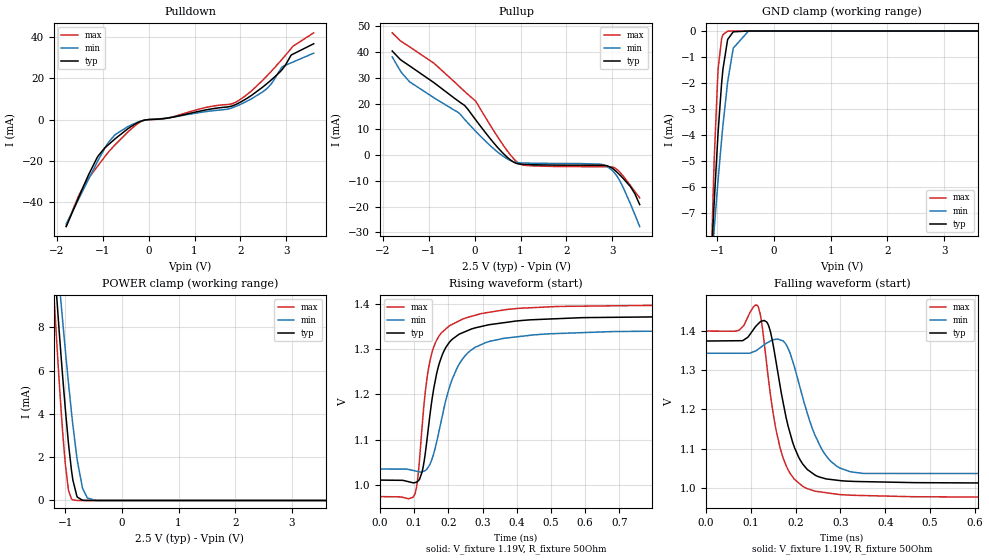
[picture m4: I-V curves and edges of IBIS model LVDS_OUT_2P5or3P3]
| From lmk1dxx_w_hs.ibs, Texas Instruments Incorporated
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|   LVDS_OUT_2P5or3P3 Model
[Model]   LVDS_OUT_2P5or3P3
Model_type   Output
Polarity   Non-Inverting
Vmeas = 1.19
Vref = 1.19
Cref = 0pF
Rref = 50
|   typ   min   max
C_comp   0.89pF   0.82pF   0.98pF
[Rac]   50   NA   NA
[Cac]   2p   NA   NA
[Voltage Range]   2.5   2.375   2.625
[Temperature Range]   45   150   -40
[Pullup Reference]   2.5   2.375   2.625
[Pulldown Reference]   -0   -0   0
[Power Clamp Reference]   2.5   2.375   2.625
[GND Clamp Reference]   0   0   0
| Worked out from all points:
|   slope of the pulldown table from 0 to 0.375 V, typ, clamps not added: 633 ohm
|   slope of the pullup table from 0 to 0.375 V, typ, clamps not added: 43.6 ohm
|   GND clamp passes 1 mA (typ) near -0.87 V on its own axis
|   POWER clamp passes 1 mA (typ) near -0.87 V on its own axis
|   falling waveform, V_fixture 1.19V, R_fixture 50Ohm: 20-80 % time 46.2ps typ, 56.5ps min, 42.8ps max; typ from 1.37 V to 1.01 V
|   rising waveform, V_fixture 1.19V, R_fixture 50Ohm: 20-80 % time 55.3ps typ, 77.9ps min, 45.5ps max; typ from 1.01 V to 1.37 V
[Pulldown]
|   Voltage   I(typ)   I(min)   I(max)
-1.8V     -51.72mA   -50.46mA   -51.57mA
-1.534V   -37.99mA   -38.69mA   -37.03mA
-1.373V   -29.73mA   -31.57mA   -30.17mA
-1.131V   -18.64mA   -20.88mA   -22.99mA
-732.4mV  -9.288mA   -7.293mA   -12.16mA
-95.76mV  -287.9uA   -343.9uA   -286.1uA
407mV     681uA      803uA      707.1uA
1.927V    7.558mA    6.599mA    8.732mA
2.553V    16.88mA    14.48mA    20.46mA
2.91V     24.09mA    25.47mA    29.14mA
3.108V    31.15mA    27.43mA    34.35mA
3.6V      36.62mA    32.09mA    41.91mA
[GND Clamp]
|   Voltage   I(typ)   I(min)   I(max)
-1.8V     -47.22mA   -32.28mA   -90.43mA
-1.103V   -8.782mA   -9.069mA   -8.722mA
-1.072V   -7.372mA   -8.153mA   -6.225mA
-1.053V   -6.556mA   -7.61mA    -4.893mA
-988.9mV  -4.055mA   -5.855mA   -1.636mA
-982.4mV  -3.827mA   -5.684mA   -1.42mA
-922.5mV  -2.008mA   -4.177mA   -294.7uA
-899.8mV  -1.477mA   -3.648mA   -144.9uA
-818.3mV  -346uA     -1.998mA   -5.222uA
-717.3mV  -29.3uA    -659.5uA   -36.6nA
-450mV    -2.386nA   -3.724uA   -6.465pA
3.6V      0A         0A         0A
[Pullup]
|   Voltage   I(typ)   I(min)   I(max)
-1.8V     40.37mA    38.09mA    47.44mA
-1.598V   36.73mA    32.02mA    44.05mA
-1.423V   34.63mA    28.45mA    42.03mA
-886.3mV  28.05mA    22.18mA    35.58mA
-335mV    20.66mA    16.2mA     26.58mA
17.64mV   13.75mA    9.286mA    20.98mA
620.3mV   653.2uA    -454.3uA   3.868mA
959.4mV   -3.453mA   -2.995mA   -3.196mA
2.889V    -4.157mA   -4.498mA   -4.529mA
3.163V    -7.669mA   -9.912mA   -6.601mA
3.397V    -12.24mA   -18.9mA    -11.81mA
3.6V      -19.23mA   -27.77mA   -16.61mA
[POWER Clamp]
|   Voltage   I(typ)   I(min)   I(max)
-1.8V     35.35mA    33.02mA    38.41mA
-1.235V   12.58mA    14.14mA    11.07mA
-1.108V   7.901mA    10.18mA    5.58mA
-1.068V   6.535mA    8.999mA    4.045mA
-1V       4.324mA    7.032mA    1.764mA
-945.7mV  2.747mA    5.536mA    547.3uA
-890.1mV  1.424mA    4.11mA     81.35uA
-863.6mV  938uA      3.477mA    28.21uA
-793.4mV  199.1uA    1.989mA    1.463uA
-694.6mV  11.18uA    577.1uA    13.83nA
-607.7mV  708.9nA    109.9uA    194.5pA
3.6V      0A         0A         0A
[Ramp]
R_load = 50
|   typ   min   max
dV/dt_r   0.218215/5.53455e-11   0.184933/7.76323e-11   0.255165/4.53755e-11
dV/dt_f   0.218303/4.60884e-11   0.1852/5.65262e-11   0.255121/4.28224e-11
[Falling Waveform]
V_fixture = 1.19V
V_fixture_min = 1.19V
V_fixture_max = 1.19V
R_fixture = 50Ohm
C_fixture = 0F
|   Time   V(typ)   V(min)   V(max)
0s        1.373V     1.342V     1.399V
74.25ps   1.374V     1.342V     1.401V
115.2ps   1.415V     1.351V     1.463V
140.8ps   1.409V     1.371V     1.265V
156.9ps   1.318V     1.378V     1.146V
179.3ps   1.177V     1.364V     1.056V
226.2ps   1.048V     1.191V     999.1mV
256.7ps   1.027V     1.102V     990.4mV
296.6ps   1.02V      1.053V     984.2mV
5ns       1.009V     1.034V     973.5mV
[Rising Waveform]
V_fixture = 1.19V
V_fixture_min = 1.19V
V_fixture_max = 1.19V
R_fixture = 50Ohm
C_fixture = 0F
|   Time   V(typ)   V(min)   V(max)
0s        1.01V      1.035V     973.5mV
102.3ps   1.005V     1.031V     978.7mV
111.4ps   1.008V     1.029V     1.019V
123.5ps   1.028V     1.029V     1.129V
138.7ps   1.106V     1.036V     1.241V
172.3ps   1.265V     1.116V     1.329V
200.4ps   1.313V     1.209V     1.351V
237.2ps   1.336V     1.274V     1.365V
366.1ps   1.36V      1.325V     1.388V
5ns       1.374V     1.343V     1.399V
